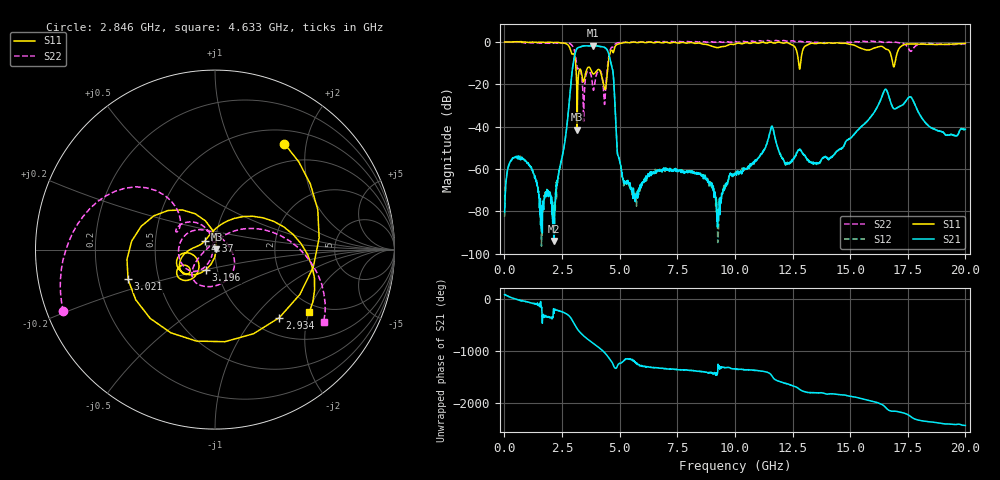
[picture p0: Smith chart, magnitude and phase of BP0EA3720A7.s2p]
! 9/17/2020 12:49:29 PM
! C:\ANRITSUVNA\DATA\MLO\SAMPLES\RAYTHEOM BP\17370_20GH_91720 .S2P
! CHANNEL.1
! TR.MEASUREMENT
! CORRECTED.DATA
# GHZ S RI R 50.0
! FREQ.GHZ  S11RE  S11IM  S31RE  S31IM  S13RE  S13IM  S33RE  S33IM
!; PortSelection: Port_13
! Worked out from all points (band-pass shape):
!   1601 points, 10 MHz to 20 GHz, reference 50 ohm
!   highest |S21| = -1.72 dB at 3.846 GHz (marker M1); lowest = -94.1 dB at 2.146 GHz (marker M2)
!   |S21| within 3 dB of the highest: 3.086 GHz to 4.498 GHz (1.412 GHz wide, 37.2 % of centre)
!   lowest |S11| = -41.4 dB at 3.158 GHz (marker M3), VSWR 1.02, Z = 50.8 + j0.182 ohm
!   |S11| at or under -10 dB: 3.089 GHz to 4.506 GHz (1.418 GHz wide, 37.3 % of centre); 12.77 GHz to 12.85 GHz (83.37 MHz wide, 0.651 % of centre); 16.85 GHz to 16.94 GHz (96.71 MHz wide, 0.572 % of centre)
!   |S22| runs from -37.6 to 0.7 dB; largest |S21 - S12| = 0.0027
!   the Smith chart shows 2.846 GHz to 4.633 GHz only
!   S11 on the Smith chart (normalised r, x): 2.846 GHz: 0.69, +1.63; 2.934 GHz: 1.31, -1.37; 3.021 GHz: 0.33, -0.15; 3.196 GHz: 0.88, -0.20; 4.37 GHz: 0.89, +0.09; 4.633 GHz: 1.74, -2.01
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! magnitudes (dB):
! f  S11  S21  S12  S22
! 10 MHz  0.0  -80.2  -82.5  0.0
! 559.7 MHz  0.1  -54.3  -54.5  -0.2
! 2.146 GHz  -0.3  -94.1  -88.4  -0.6
! 2.846 GHz  -3.0  -24.5  -24.4  -0.8
! 2.934 GHz  -5.7  -14.5  -14.5  -1.6
! 3.021 GHz  -5.8  -8.0  -7.9  -3.4
! 3.158 GHz  -41.4  -3.0  -3.0  -12.4
! 3.196 GHz  -18.2  -2.7  -2.7  -12.6
! 3.346 GHz  -14.6  -2.1  -2.1  -15.6
! 3.846 GHz  -15.0  -1.7  -1.7  -22.0
! 4.37 GHz  -22.5  -2.7  -2.7  -26.2
! 4.633 GHz  -4.0  -10.4  -10.4  -2.8
! 4.933 GHz  -1.0  -53.8  -53.9  -0.4
! 5.195 GHz  -0.3  -65.6  -68.1  -0.2
! 6.682 GHz  -0.1  -60.7  -61.0  0.0
! 8.618 GHz  -1.0  -62.7  -62.8  0.2
! 9.293 GHz  -2.6  -79.2  -87.3  0.1
! 10.01 GHz  -1.0  -62.2  -62.0  0.2
! 11.6 GHz  -0.2  -39.8  -39.8  0.2
! 13.34 GHz  -0.6  -57.1  -57.2  -0.2
! 16.68 GHz  -4.0  -25.6  -25.6  -0.1
! 20 GHz  -0.7  -41.3  -41.1  -0.8
